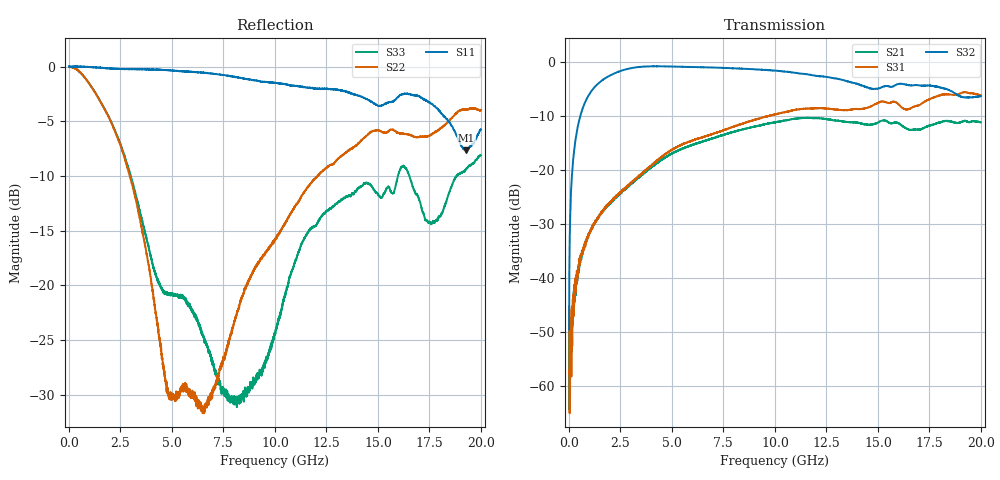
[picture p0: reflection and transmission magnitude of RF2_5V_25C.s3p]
!Keysight Technologies,N5244B,MY57181157,A.18.40.03
!Date: Friday, December 19, 2025 13:28:36
!Correction: S11(C  3-Port  )
!S12(C  3-Port  )
!S13(C  3-Port  )
!S21(C  3-Port  )
!S22(C  3-Port  )
!S23(C  3-Port  )
!S31(C  3-Port  )
!S32(C  3-Port  )
!S33(C  3-Port  )
!S3P File: Measurements: <S11,S12,S13>,
!<S21,S22,S23>,
!<S31,S32,S33>:
# Hz S  dB  R 50
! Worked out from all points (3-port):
!   3999 points, 10 MHz to 20 GHz, reference 50 ohm
!   strongest paths, dB at 10 MHz, 5.005 GHz, 10.01 GHz, 15.01 GHz, 20 GHz:
!     S32: -49.5, -0.8, -1.6, -4.9, -6.3
!     S31: -45.3, -16.2, -9.7, -7.5, -6.1
!     S21: -46.3, -16.9, -11.1, -11.2, -11.1
!   lowest |S11| = -7.6 dB at 19.29 GHz (marker M1), VSWR 2.42, Z = 20.8 + j2.82 ohm
!   |S11| at or under -10 dB: nowhere
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1e7  0.03 -0.1  -50.10 -91.7  -43.23 102.8
     -46.32 69.9  -0.04 -0.6  -48.92 101.3
     -45.26 -135.5  -49.46 97.3  0.00 -0.2
1.35e8  -0.02 -1.2  -50.70 91.3  -50.88 111.7
        -51.87 130.8  -0.05 -6.0  -21.86 87.8
        -45.78 99.5  -21.73 87.1  -0.06 -5.8
3.2e8  -0.01 -2.7  -40.93 87.0  -40.82 89.6
       -40.21 97.8  -0.19 -13.9  -14.38 76.8
       -42.44 98.1  -14.40 76.8  -0.19 -13.7
1.33e9  -0.08 -10.9  -29.36 78.9  -29.12 82.6
        -29.39 78.7  -2.57 -49.8  -4.30 39.6
        -29.21 82.4  -4.31 39.5  -2.54 -46.4
4.915e9  -0.34 -27.9  -17.05 55.4  -16.43 69.4
         -17.10 55.6  -30.45 -140.8  -0.79 -24.0
         -16.39 69.2  -0.81 -23.9  -20.71 -60.3
7.92e9  -0.90 -55.8  -12.97 24.1  -12.04 44.4
        -12.99 24.2  -24.12 91.1  -1.14 -54.8
        -12.03 44.3  -1.11 -54.8  -30.55 -39.6
1.0005e10  -1.48 -76.7  -11.11 0.4  -9.69 25.7
           -11.11 0.1  -15.83 97.6  -1.57 -75.1
           -9.69 25.6  -1.57 -75.2  -24.52 -123.0
1.623e10  -2.54 -155.5  -11.93 -71.8  -8.56 -29.2
          -11.94 -72.0  -6.14 78.0  -4.05 -121.0
          -8.59 -29.2  -4.07 -121.0  -9.06 -179.9
1.929e10  -7.64 172.2  -10.89 -94.9  -5.58 -51.7
          -10.92 -94.8  -3.92 35.7  -6.54 -146.5
          -5.58 -51.6  -6.54 -146.3  -9.33 135.0
2e10  -5.74 163.1  -11.10 -105.8  -6.12 -61.0
      -11.13 -105.8  -3.99 45.8  -6.25 -147.4
      -6.12 -60.9  -6.27 -147.3  -8.10 145.0
